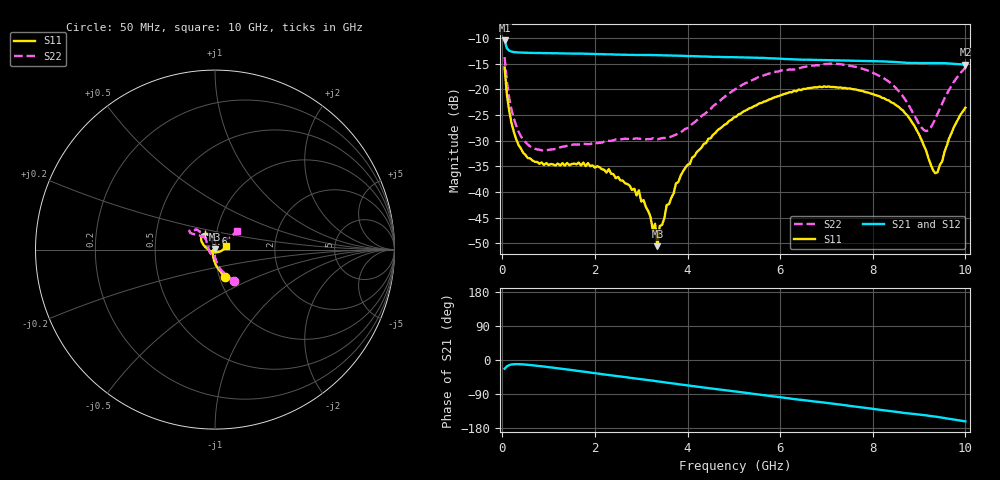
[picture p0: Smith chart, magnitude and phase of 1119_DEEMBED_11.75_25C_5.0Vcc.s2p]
!Hittite Microwave Corp.
!Digital Attenuator/PhaseShifter Rev 1.4.0
!Filename: C:\DATA\DATA\1119_DEEMBED_11.75_25C_5.0Vcc.s2p
!VNA ID: Agilent Technologies,N5224A,MY51441122,A.10.45.03
!Device type:
!2 Port Calibration.
!Temp(C): 25
!Lot Number:
!Serial Number:
!Operator:
!Misc:
!Attenuator:  11.750
# GHZ S DB R 50.0
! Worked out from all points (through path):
!   200 points, 50 MHz to 10 GHz, reference 50 ohm
!   highest |S21| = -10.48 dB at 50 MHz (marker M1); lowest = -15.2 dB at 10 GHz (marker M2)
!   group delay of S21, straight-line fit = 43.1 ps
!   lowest |S11| = -50.5 dB at 3.35 GHz (marker M3), VSWR 1.01, Z = 49.7 + j0.127 ohm
!   |S11| at or under -10 dB: start of sweep to end of sweep
!   |S22| runs from -31.9 to -13.7 dB; largest |S21 - S12| = 0.00058
!   S11 on the Smith chart (normalised r, x): 50 MHz: 1.06, -0.34; 6.6 GHz: 0.88, +0.16; 10 GHz: 1.13, +0.05
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0.05  -15.74 -71.1  -10.48 -22.9  -10.48 -23.0  -13.71 -59.0
0.1  -21.09 -86.4  -12.04 -16.8  -12.03 -16.8  -18.54 -73.8
0.2  -26.61 -101.1  -12.65 -11.8  -12.65 -11.8  -24.00 -84.7
0.45  -32.35 -121.9  -12.86 -11.6  -12.86 -11.6  -29.75 -93.6
0.85  -34.24 -140.3  -12.93 -16.6  -12.94 -16.6  -31.86 -100.8
1.75  -34.27 -148.7  -13.06 -30.7  -13.06 -30.7  -30.62 -112.4
2.95  -39.66 -139.5  -13.30 -49.7  -13.30 -49.8  -29.61 -149.5
3.25  -47.40 -167.1  -13.32 -54.7  -13.33 -54.7  -29.53 -163.8
3.3  -46.17 175.6  -13.34 -55.5  -13.34 -55.6  -29.68 -166.5
3.35  -50.53 154.7  -13.35 -56.3  -13.36 -56.4  -29.73 -168.6
3.4  -46.61 153.4  -13.35 -57.1  -13.35 -57.1  -29.60 -170.8
3.75  -38.32 92.8  -13.42 -63.0  -13.43 -63.0  -28.80 170.4
4.1  -33.29 83.9  -13.53 -68.7  -13.54 -68.7  -26.75 151.5
5.05  -25.33 93.0  -13.75 -83.4  -13.77 -83.4  -19.86 128.7
6.6  -19.79 121.8  -14.24 -107.2  -14.26 -107.3  -15.49 139.7
6.7  -19.68 123.6  -14.25 -108.7  -14.26 -108.8  -15.35 140.2
7.65  -20.07 142.0  -14.43 -123.2  -14.44 -123.2  -15.65 146.0
8.35  -22.18 153.5  -14.62 -134.5  -14.62 -134.5  -18.53 138.2
8.75  -25.12 165.3  -14.85 -140.6  -14.84 -140.6  -22.69 126.5
9.1  -30.89 -166.1  -14.88 -145.3  -14.89 -145.3  -27.90 97.8
9.35  -36.34 -98.8  -14.86 -149.4  -14.88 -149.4  -25.73 58.2
10  -23.58 18.7  -15.19 -162.0  -15.20 -162.0  -15.78 40.2
